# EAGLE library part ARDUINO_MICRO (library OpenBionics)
Breakout Board for Arduino Micro
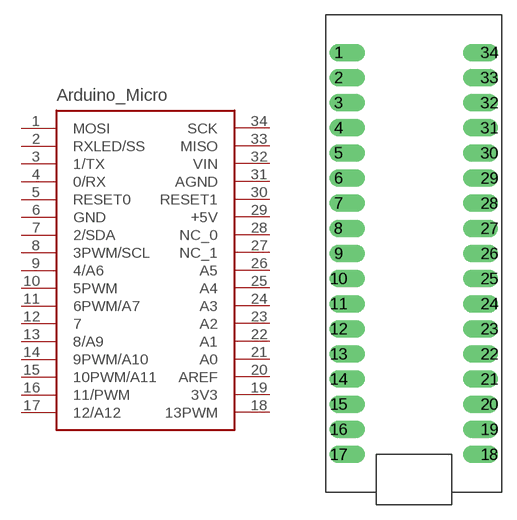
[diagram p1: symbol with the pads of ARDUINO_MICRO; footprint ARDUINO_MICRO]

Designator prefix -

## ARDUINO_MICROARDUINO_BOARD  [ARDUINO_MICRO]
1  MOSI
2  RXLED/SS
3  1/TX
4  0/RX
5  RESET0
6  GND
7  2/SDA
8  3PWM/SCL
9  4/A6
10  5PWM
11  6PWM/A7
12  7
13  8/A9
14  9PWM/A10
15  10PWM/A11
16  11/PWM
17  12/A12
18  13PWM
19  3V3
20  AREF
21  A0
22  A1
23  A2
24  A3
25  A4
26  A5
27  NC_1  nc
28  NC_0  nc
29  +5V
30  RESET1
31  AGND
32  VIN
33  MISO
34  SCK

## Footprint ARDUINO_MICRO (pad centres in mm)
Breakout Board for Arduino micro
drill 1 pad 1.778 offset: 1 -7.62,20.32; 2 -7.62,17.78; 3 -7.62,15.24; 4 -7.62,12.7; 5 -7.62,10.16; 6 -7.62,7.62; 7 -7.62,5.08; 8 -7.62,2.54; 9 -7.62,0; 10 -7.62,-2.54; 11 -7.62,-5.08; 12 -7.62,-7.62; 13 -7.62,-10.16; 14 -7.62,-12.7; 15 -7.62,-15.24; 16 -7.62,-17.78; 17 -7.62,-20.32; 18 7.62,-20.32; 19 7.62,-17.78; 20 7.62,-15.24; 21 7.62,-12.7; 22 7.62,-10.16; 23 7.62,-7.62; 24 7.62,-5.08; 25 7.62,-2.54; 26 7.62,0; 27 7.62,2.54; 28 7.62,5.08; 29 7.62,7.62; 30 7.62,10.16; 31 7.62,12.7; 32 7.62,15.24; 33 7.62,17.78; 34 7.62,20.32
